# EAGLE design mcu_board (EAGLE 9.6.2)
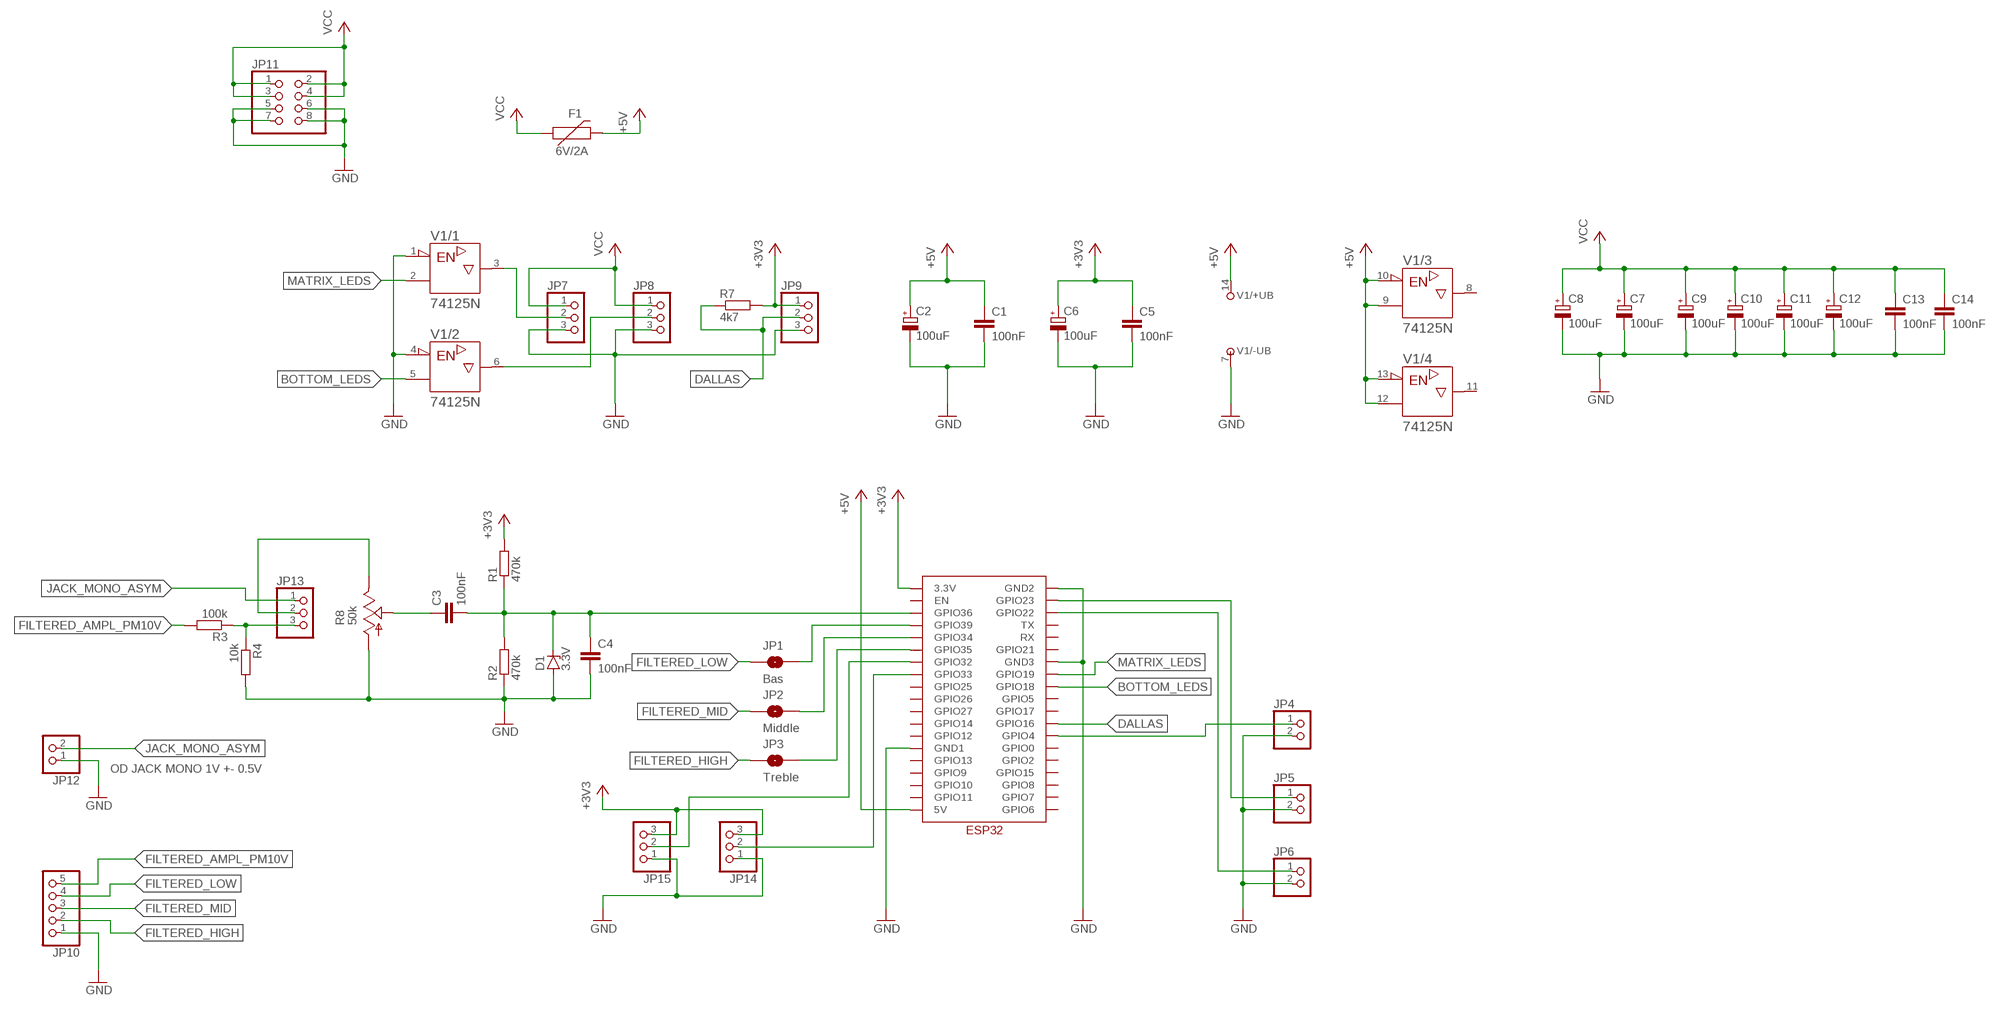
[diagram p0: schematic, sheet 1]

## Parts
C1  100nF  C-EU025-025X050  [C025-025X050]
C2  100uF  CPOL-EUE2.5-7  [E2,5-7]
C3  100nF  C-EU025-025X050  [C025-025X050]
C4  100nF  C-EU025-025X050  [C025-025X050]
C5  100nF  C-EU025-025X050  [C025-025X050]
C6  100uF  CPOL-EUE2.5-7  [E2,5-7]
C7  100uF  CPOL-EUE2.5-7  [E2,5-7]
C8  100uF  CPOL-EUE2.5-7  [E2,5-7]
C9  100uF  CPOL-EUE2.5-7  [E2,5-7]
C10  100uF  CPOL-EUE2.5-7  [E2,5-7]
C11  100uF  CPOL-EUE2.5-7  [E2,5-7]
C12  100uF  CPOL-EUE2.5-7  [E2,5-7]
C13  100nF  C-EU025-025X050  [C025-025X050]
C14  100nF  C-EU025-025X050  [C025-025X050]
D1  3.3V  ZENER-DIODEDO34-7  [DO34Z7]
F1  6V/2A  PPTC_6V2A  [1210]
JP1  Bas  JUMPER-SMT_2_NO_NO-SILK  [SMT-JUMPER_2_NO_NO-SILK]
JP2  Middle  JUMPER-SMT_2_NO_NO-SILK  [SMT-JUMPER_2_NO_NO-SILK]
JP3  Treble  JUMPER-SMT_2_NO_NO-SILK  [SMT-JUMPER_2_NO_NO-SILK]
JP4  PINHD-1X2  [1X02]
JP5  PINHD-1X2  [1X02]
JP6  PINHD-1X2  [1X02]
JP7  PINHD-1X3  [1X03]
JP8  PINHD-1X3  [1X03]
JP9  PINHD-1X3  [1X03]
JP10  PINHD-1X5  [1X05]
JP11  PINHD-2X4  [2X04]
JP12  PINHD-1X2  [1X02]
JP13  PINHD-1X3  [1X03]
JP14  PINHD-1X3  [1X03]
JP15  PINHD-1X3  [1X03]
R1  470k  R-EU_0207/7  [0207/7]
R2  470k  R-EU_0207/7  [0207/7]
R3  100k  R-EU_0207/7  [0207/7]
R4  10k  R-EU_0207/7  [0207/7]
R7  4k7  R-EU_0207/7  [0207/7]
R8  50k  TRIM_US-CA6V  [CA6V]
U$2  ESP32  [ESP32]
V1  74125N  [DIL14]

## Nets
+3V3: C5.1 C6.+ JP9.1 JP14.3 JP15.3 R1.2 R7.2 U$2.3.3V
+5V: C1.1 C2.+ F1.2 U$2.5V V1.9(/3:A) V1.10(/3:!G) V1.12(/4:A) V1.13(/4:!G) V1.14(/+UB:+UB)
BOTTOM_LEDS: U$2.GPIO18 V1.5(/2:A)
DALLAS: JP9.2 R7.1 U$2.GPIO16
FILTERED_AMPL_PM10V: JP10.5 R3.2
FILTERED_HIGH: JP3.1 JP10.2
FILTERED_LOW: JP1.1 JP10.4
FILTERED_MID: JP2.1 JP10.3
GND: C1.2 C2.- C4.2 C5.2 C6.- C7.- C8.- C9.- C10.- C11.- C12.- C13.2 C14.2 D1.A JP4.2 JP5.2 JP6.2 JP7.3 JP8.3 JP9.3 JP10.1 JP11.5 JP11.6 JP11.7 JP11.8 JP12.1 JP14.1 JP15.1 R2.1 R4.2 R8.A U$2.GND1 U$2.GND2 U$2.GND3 V1.1(/1:!G) V1.4(/2:!G) V1.7(/-UB:-UB)
JACK_MONO_ASYM: JP12.2 JP13.1
MATRIX_LEDS: U$2.GPIO19 V1.2(/1:A)
N$1: C3.1 R8.S
N$2: JP1.2 U$2.GPIO39
N$3: JP13.2 R8.E
N$4: C3.2 C4.1 D1.C R1.1 R2.2 U$2.GPIO36
N$5: JP2.2 U$2.GPIO34
N$6: JP8.2 V1.6(/2:Y)
N$7: JP3.2 U$2.GPIO35
N$8: JP7.2 V1.3(/1:Y)
N$9: JP15.2 U$2.GPIO32
N$10: JP13.3 R3.1 R4.1
N$14: JP14.2 U$2.GPIO33
N$16: JP4.1 U$2.GPIO4
N$17: JP5.1 U$2.GPIO23
N$18: JP6.1 U$2.GPIO22
VCC: C7.+ C8.+ C9.+ C10.+ C11.+ C12.+ C13.1 C14.1 F1.1 JP7.1 JP8.1 JP11.1 JP11.2 JP11.3 JP11.4
Unconnected: U$2.EN U$2.GPIO0 U$2.GPIO2 U$2.GPIO5 U$2.GPIO6 U$2.GPIO7 U$2.GPIO8 U$2.GPIO9 U$2.GPIO10 U$2.GPIO11 U$2.GPIO12 U$2.GPIO13 U$2.GPIO14 U$2.GPIO15 U$2.GPIO17 U$2.GPIO21 U$2.GPIO25 U$2.GPIO26 U$2.GPIO27 U$2.RX U$2.TX V1.8(/3:Y) V1.11(/4:Y)

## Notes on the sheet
- OD JACK MONO 1V +- 0.5V

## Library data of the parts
C1 C3-C5 C13 C14 = rcl:C-EU: CAPACITOR, European symbol; SPICEPREFIX: C
C2 C6-C12 = rcl:CPOL-EU: POLARIZED CAPACITOR, European symbol; SPICEPREFIX: C
D1 = diode:ZENER-DIODE: Z-Diode
F1 = SparkFun-Fuses:PPTC: Resettable Fuse PPTC; PROD_ID: RES-14313
JP1-JP3 = SparkFun-Jumpers:JUMPER-SMT_2_NO: Normally open jumper
JP4-JP6 JP12 = pinhead:PINHD-1X2: PIN HEADER
JP7-JP9 JP13-JP15 = pinhead:PINHD-1X3: PIN HEADER
JP10 = pinhead:PINHD-1X5: PIN HEADER
JP11 = pinhead:PINHD-2X4: PIN HEADER
R1-R4 R7 = rcl:R-EU_: RESISTOR, European symbol; SPICEPREFIX: R
R8 = pot:TRIM_US-: POTENTIOMETER
U$2 = ESP32:ESP32
V1 = 74ttl-din:74*125: Quad bus BUFFER, 3-state

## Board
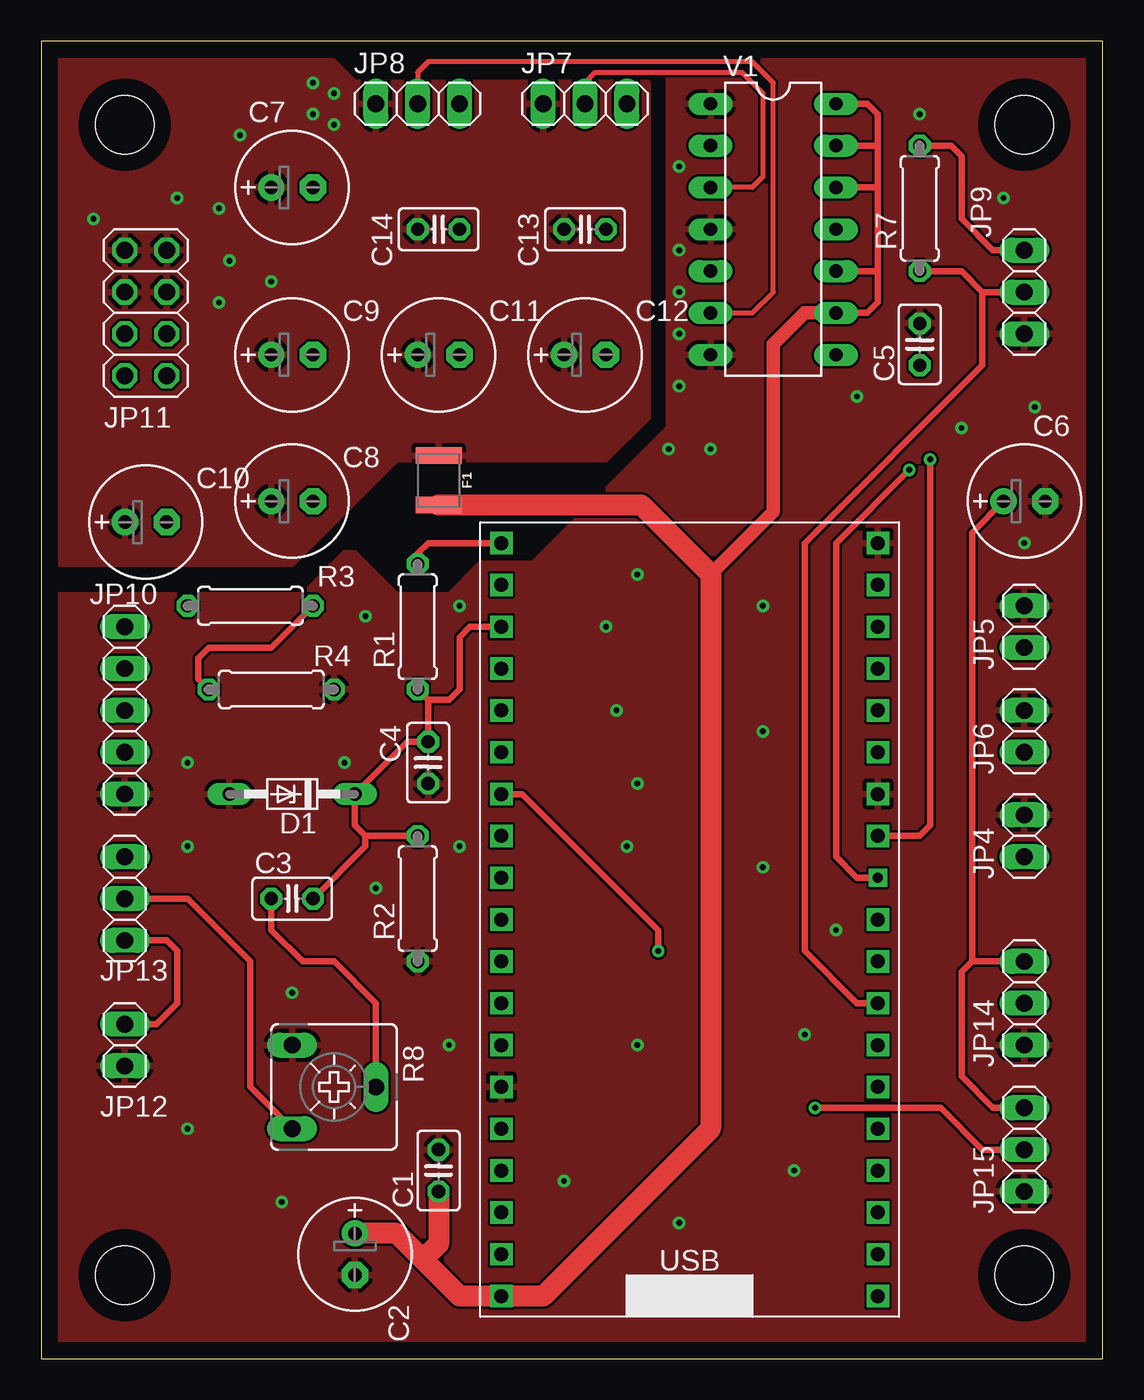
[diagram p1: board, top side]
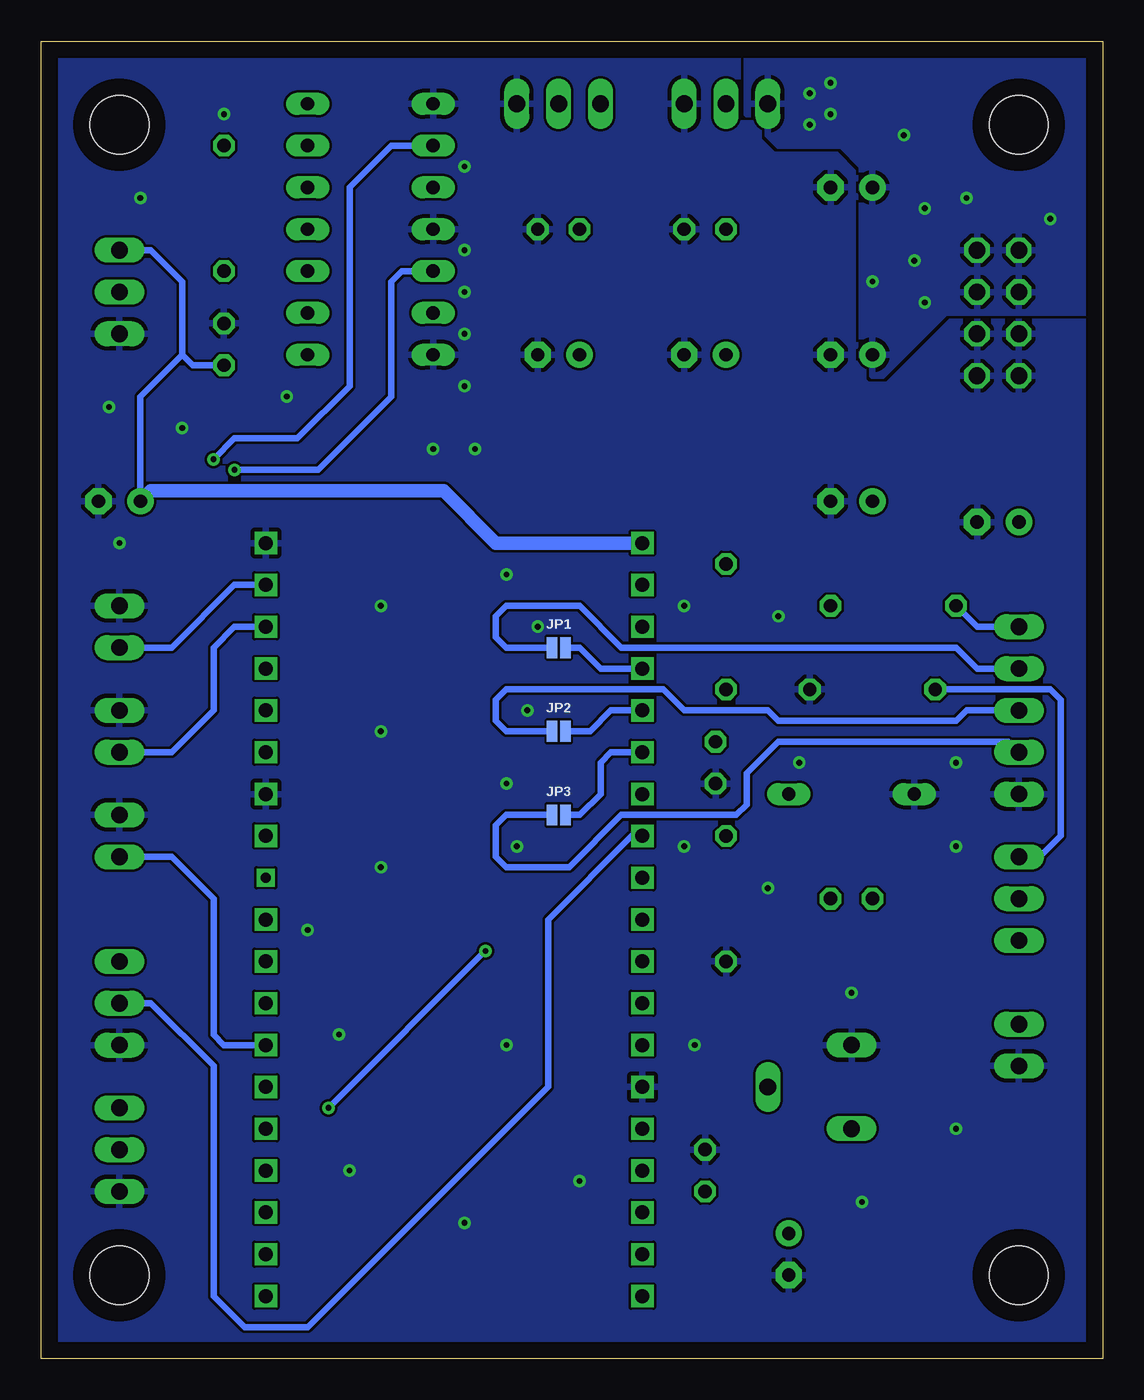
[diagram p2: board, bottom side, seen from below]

Size 64.44 x 80 mm. Coordinates in mm from the lower left corner, seen from the top.
Outline: 0,0 64.44,0 64.44,80 0,80 0,0
Copper layers (1*16): Top 0.035mm / dielectric 1.5mm / Bottom 0.035mm
Design rules "default *": minimum track width 6mil, minimum drill 0.35mm, track to track 6mil, track to pad 6mil, pad to pad 6mil, via to via 6mil, smd to smd 6mil, copper to edge 40mil, drill to drill 6mil, minimum pad ring 10mil, minimum via ring 8mil, stop-mask expansion 4mil, vias tented up to drill 16mil, thermal gap 10mil
Holes 3.56 mm at 5.08,74.93 59.69,74.93 59.69,5.08 5.08,5.08

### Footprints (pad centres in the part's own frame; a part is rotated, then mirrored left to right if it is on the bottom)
C025-025X050 = drill 0.813 octagon: 1 -1.27,0; 2 1.27,0
E2,5-7 = drill 0.813 pad 1.6: + -1.27,0 | drill 0.813 pad 1.6 octagon: - 1.27,0
DO34Z7 = drill 0.813 long: A 3.81,0; C -3.81,0
1210 = smd 1 x 2.8: 1 -1.5,0; 2 1.5,0
SMT-JUMPER_2_NO_NO-SILK = smd 0.635 x 1.27: 1 -0.406,0; 2 0.406,0
1X02 = drill 1.016 long: 1 -1.27,0; 2 1.27,0
1X03 = drill 1.016 long: 1 -2.54,0; 2 0,0; 3 2.54,0
1X05 = drill 1.016 long: 1 -5.08,0; 2 -2.54,0; 3 0,0; 4 2.54,0; 5 5.08,0
2X04 = drill 1.016 octagon: 1 -3.81,-1.27; 2 -3.81,1.27; 3 -1.27,-1.27; 4 -1.27,1.27; 5 1.27,-1.27; 6 1.27,1.27; 7 3.81,-1.27; 8 3.81,1.27
0207/7 = drill 0.813 octagon: 1 -3.81,0; 2 3.81,0
CA6V = drill 1.016 long: A -2.54,-2.54; E 2.54,-2.54; S 0,2.54
ESP32 = drill 0.85 square: 3.3V 1.27,46.99; 5V 1.27,1.27; EN 1.27,44.45; GND1 1.27,13.97; GND2 24.13,46.99; GND3 24.13,31.75; GPIO0 24.13,13.97; GPIO2 24.13,11.43; GPIO4 24.13,16.51; GPIO5 24.13,24.13; GPIO6 24.13,1.27; GPIO7 24.13,3.81; GPIO8 24.13,6.35; GPIO9 1.27,8.89; GPIO10 1.27,6.35; GPIO11 1.27,3.81; GPIO12 1.27,16.51; GPIO13 1.27,11.43; GPIO14 1.27,19.05; GPIO15 24.13,8.89; GPIO16 24.13,19.05; GPIO17 24.13,21.59; GPIO19 24.13,29.21; GPIO21 24.13,34.29; GPIO22 24.13,41.91; GPIO23 24.13,44.45; GPIO25 1.27,26.67; GPIO26 1.27,24.13; GPIO27 1.27,21.59; GPIO32 1.27,31.75; GPIO33 1.27,29.21; GPIO34 1.27,36.83; GPIO35 1.27,34.29; GPIO36 1.27,41.91; GPIO39 1.27,39.37; RX 24.13,36.83; TX 24.13,39.37 | drill 0.6 square: GPIO18 24.13,26.67
DIL14 = drill 0.813 long: 1 -7.62,-3.81; 2 -5.08,-3.81; 3 -2.54,-3.81; 4 0,-3.81; 5 2.54,-3.81; 6 5.08,-3.81; 7 7.62,-3.81; 8 7.62,3.81; 9 5.08,3.81; 10 2.54,3.81; 11 0,3.81; 12 -2.54,3.81; 13 -5.08,3.81; 14 -7.62,3.81

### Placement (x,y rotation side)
C1  24.13,11.43 90 top
C2  19.05,6.35 270 top
C3  15.24,27.94 0 top
C4  23.5,36.2 270 top
C5  53.34,61.59 90 top
C6  59.69,52.07 0 top
C7  15.24,71.12 0 top
C8  15.24,52.07 0 top
C9  15.24,60.96 0 top
C10  6.35,50.8 0 top
C11  24.13,60.96 0 top
C12  33.02,60.96 0 top
C13  33.02,68.58 0 top
C14  24.13,68.58 0 top
D1  15.24,34.29 180 top
F1  24.13,53.34 270 top
JP1  33.02,43.18 0 bottom
JP2  33.02,38.1 0 bottom
JP3  33.02,33.02 0 bottom
JP4  59.69,31.75 90 top
JP5  59.69,44.45 90 top
JP6  59.69,38.1 90 top
JP7  33.02,76.2 0 top
JP8  22.86,76.2 0 top
JP9  59.69,64.77 270 top
JP10  5.08,39.37 90 top
JP11  6.35,63.5 270 top
JP12  5.08,19.05 90 top
JP13  5.08,27.94 90 top
JP14  59.69,21.59 90 top
JP15  59.69,12.7 90 top
R1  22.86,44.45 90 top
R2  22.86,27.94 90 top
R3  12.7,45.72 180 top
R4  13.97,40.64 0 top
R7  53.34,69.85 90 top
R8  17.78,16.51 270 top
U$2  26.67,2.54 0 top
V1  44.45,68.58 270 top

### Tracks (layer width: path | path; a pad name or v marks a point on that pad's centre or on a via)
+3V3
  Top 0.406: JP9.1 57.78,67.31 55.88,69.22 55.88,73.03 55.24,73.66 R7.2 | JP14.3 56.52,24.13 | 56.52,24.13 55.88,23.5 55.88,17.14 57.78,15.24 JP15.3 | 56.52,24.13 56.52,50.16 C6.+ | R1.2 22.86,48.9 23.5,49.53 U$2.3.3V
  Bottom 0.406: JP9.1 57.78,67.31 55.88,65.41 55.88,60.96 | 55.88,60.96 55.24,60.33 C5.1 | 55.88,60.96 58.42,58.42 C6.+
  Bottom 0.813: C6.+ 57.78,52.7 40.01,52.7 36.83,49.53 U$2.3.3V
+5V
  Top 0.406: 50.8,66.04 50.8,64.14 50.16,63.5 V1.9 | 50.8,66.04 50.8,71.12 | 50.8,71.12 50.8,73.66 | 50.8,73.66 50.8,75.56 50.16,76.2 V1.14 | V1.13 50.8,73.66 | V1.12 50.8,71.12 | V1.10 50.8,66.04
  Top 0.813: V1.9 46.35,63.5 44.45,61.59 44.45,51.44 40.64,47.62
  Top 1.27: F1.2 36.42,51.84 40.64,47.62 40.64,13.97 30.48,3.81 U$2.5V 25.4,3.81 23.18,6.03 | 23.18,6.03 21.59,7.62 C2.+ | C1.1 24.13,6.99 23.18,6.03
BOTTOM_LEDS  (via drill 0.35)
  Top 0.406: U$2.GPIO18 49.53,29.21 48.26,30.48 48.26,49.53 v52.7,53.98
  Bottom 0.406: V1.5 42.55,66.04 43.18,65.41 43.18,58.42 47.62,53.98 v52.7,53.98
DALLAS
  Top 0.406: JP9.2 57.15,64.77 | 57.15,64.77 55.88,66.04 R7.1 | U$2.GPIO16 49.53,21.59 46.35,24.77 46.35,49.53 57.15,60.33 57.15,64.77
FILTERED_AMPL_PM10V
  Bottom 0.406: JP10.5 7.62,44.45 R3.2
FILTERED_HIGH
  Bottom 0.406: JP10.2 5.71,37.47 19.68,37.47 21.59,35.56 21.59,33.66 22.23,33.02 29.21,33.02 32.38,29.84 36.2,29.84 36.83,30.48 36.83,32.38 36.2,33.02 JP3.1
FILTERED_LOW
  Bottom 0.406: JP10.4 7.62,41.91 8.89,43.18 29.21,43.18 31.75,45.72 36.2,45.72 36.83,45.09 36.83,43.81 36.2,43.18 JP1.1
FILTERED_MID
  Bottom 0.406: JP10.3 8.26,39.37 8.89,38.73 19.68,38.73 20.32,39.37 25.4,39.37 26.67,40.64 36.2,40.64 36.83,40.01 36.83,38.73 36.2,38.1 JP2.1
GND  (via drill 0.35)
  other vias: 40.64,55.24 55.88,56.52 60.33,57.78 58.42,70.48 53.34,75.56 8.89,31.11 20.32,28.57 25.4,31.11 18.41,36.2 8.89,36.2 19.68,45.09 25.4,45.72 36.2,47.62 34.29,44.45 34.92,39.37 36.2,34.92 35.56,31.11 43.81,29.84 43.81,38.1 43.81,45.72 8.89,13.97 14.61,9.53 31.75,10.79 15.24,22.23 24.77,19.05 45.72,11.43 46.35,19.68 48.26,26.04 38.73,8.26 36.2,19.05 49.53,58.42 59.69,49.53 38.73,67.31 38.73,72.39 38.73,62.23 38.73,64.77 38.73,59.05 38.1,55.24
  pour Bottom (rank 2): -0.64,80.64 64.77,80.64 65.41,80.01 65.41,-0.64 -0.64,-0.64
  pour Top: -0.64,46.35 15.24,46.35 15.88,46.35 18.41,48.9 19.05,48.9 21.59,46.35 24.77,46.35 26.67,48.26 29.84,48.26 38.1,56.52 38.1,80.64 66.67,80.64 66.67,0 64.14,-2.54 62.87,-3.81 -1.91,-3.81 -1.91,46.35
JACK_MONO_ASYM
  Top 0.406: JP12.2 6.99,20.32 8.26,21.59 8.26,24.77 7.62,25.4 JP13.1
MATRIX_LEDS  (via drill 0.35)
  Top 0.406: U$2.GPIO19 53.34,31.75 53.98,32.38 v53.98,54.61
  Bottom 0.406: V1.2 43.18,73.66 45.72,71.12 45.72,59.05 48.9,55.88 52.7,55.88 v53.98,54.61
N$1
  Top 0.406: C3.1 13.97,26.04 15.88,24.13 17.78,24.13 20.32,21.59 R8.S
N$2
  Bottom 0.406: U$2.GPIO39 30.48,41.91 31.75,43.18 JP1.2
N$3
  Top 0.406: JP13.2 8.89,27.94 12.7,24.13 12.7,16.51 R8.E
N$4
  Top 0.406: R1.1 23.5,40.01 | 23.5,40.01 C4.1 22.23,37.47 D1.C 19.05,32.38 19.68,31.75 | 23.5,40.01 24.77,40.01 25.4,40.64 25.4,43.81 26.04,44.45 U$2.GPIO36 | R2.2 19.68,31.75 | C3.2 19.68,31.11 19.68,31.75
N$5
  Bottom 0.406: JP2.2 31.11,38.1 29.84,39.37 U$2.GPIO34
N$6
  Top 0.305: V1.6 43.18,63.5 44.45,64.77 44.45,77.47 43.18,78.74 23.5,78.74 22.86,78.11 JP8.2
N$7
  Bottom 0.406: JP3.2 31.75,33.02 30.48,34.29 30.48,36.2 29.84,36.83 U$2.GPIO35
N$8
  Top 0.305: JP7.2 33.02,77.47 33.66,78.11 42.55,78.11 43.81,76.83 43.81,71.75 43.18,71.12 V1.3
N$9  (via drill 0.35)
  Top 0.406: U$2.GPIO32 29.21,34.29 37.47,26.04 v37.47,24.77 | v46.99,15.24 54.61,15.24 57.15,12.7 JP15.2
  Bottom 0.406: v37.47,24.77 v46.99,15.24
N$10
  Top 0.406: R3.1 13.97,43.18 10.16,43.18 9.53,42.55 9.53,41.27 R4.1
  Bottom 0.406: R4.1 3.17,40.64 2.54,40.01 2.54,31.75 3.81,30.48 JP13.3
N$14
  Bottom 0.406: JP14.2 57.78,21.59 53.98,17.78 53.98,3.81 52.07,1.91 48.26,1.91 33.66,16.51 33.66,26.67 28.57,31.75 U$2.GPIO33
N$16
  Bottom 0.406: JP4.1 56.52,30.48 53.98,27.94 53.98,19.68 53.34,19.05 U$2.GPIO4
N$17
  Bottom 0.406: U$2.GPIO23 52.7,46.99 56.52,43.18 JP5.1
N$18
  Bottom 0.406: JP6.1 56.52,36.83 53.98,39.37 53.98,43.18 52.7,44.45 U$2.GPIO22
VCC  (via drill 0.35)
  other vias: 8.26,70.48 11.43,66.67 3.17,69.22 13.97,65.41 12.06,74.3 17.78,74.93 17.78,76.83 16.51,77.47 16.51,75.56 10.79,69.85 10.79,64.14
  pour Top: 0,48.26 15.24,48.26 21.59,54.61 34.29,54.61 36.83,57.15 36.83,77.47 19.05,77.47 15.24,81.28 -1.27,81.28 -1.27,48.26
  pour Bottom: 0,63.5 9.53,63.5 13.34,59.69 13.97,59.69 14.61,60.33 14.61,66.04 14.61,72.39 15.88,73.66 19.68,73.66 21.59,75.56 21.59,80.64 -0.64,80.64 -0.64,64.14

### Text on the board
tValues: LEDS > | FRONT | BOT | PWR | PWR | 3V3 | PWR | S | 3V3 | AMP | L | M | H | M | J | SWITCH | JACK | AMPLIFIED
bValues: HOT | LOW | MID | HIGH

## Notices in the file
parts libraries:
SparkFun-Jumpers: Licensing: Creative Commons ShareAlike 4.0 International - https://creativecommons.org/licenses/by-sa/4.0
